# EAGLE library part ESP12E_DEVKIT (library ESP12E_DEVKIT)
ESP12E DEVKIT BOARD
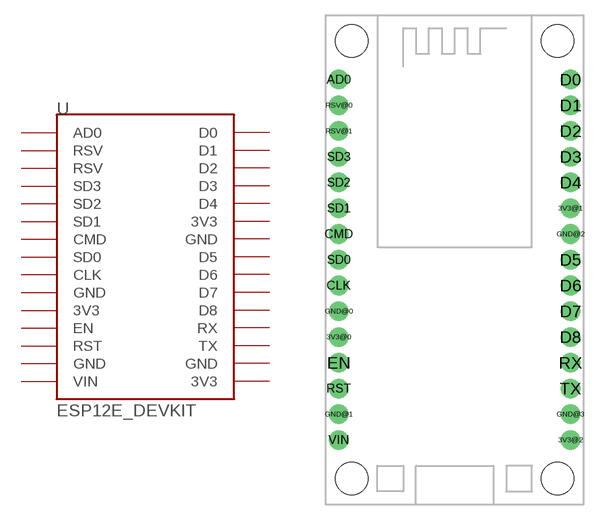
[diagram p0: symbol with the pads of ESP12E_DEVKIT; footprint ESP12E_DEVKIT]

Designator prefix -

## ESP12E_DEVKIT  [ESP12E_DEVKIT]
3V3@0  3V3
3V3@1  3V3
3V3@2  3V3
AD0  AD0
CLK  CLK
CMD  CMD
D0  D0
D1  D1
D2  D2
D3  D3
D4  D4
D5  D5
D6  D6
D7  D7
D8  D8
EN  EN
GND@0  GND
GND@1  GND
GND@2  GND
GND@3  GND
RST  RST
RSV@0  RSV
RSV@1  RSV
RX  RX
SD0  SD0
SD1  SD1
SD2  SD2
SD3  SD3
TX  TX
VIN  VIN

## Footprint ESP12E_DEVKIT (pad centres in mm)
ESP12E_DEVKIT
drill 0.8 pad 1.93: 3V3@0 -11.43,-7.62; 3V3@1 11.43,5.08; 3V3@2 11.43,-17.78; AD0 -11.43,17.78; CLK -11.43,-2.54; CMD -11.43,2.54; D0 11.43,17.78; D1 11.43,15.24; D2 11.43,12.7; D3 11.43,10.16; D4 11.43,7.62; D5 11.43,0; D6 11.43,-2.54; D7 11.43,-5.08; D8 11.43,-7.62; EN -11.43,-10.16; GND@0 -11.43,-5.08; GND@1 -11.43,-15.24; GND@2 11.43,2.54; GND@3 11.43,-15.24; RST -11.43,-12.7; RSV@0 -11.43,15.24; RSV@1 -11.43,12.7; RX 11.43,-10.16; SD0 -11.43,0; SD1 -11.43,5.08; SD2 -11.43,7.62; SD3 -11.43,10.16; TX 11.43,-12.7; VIN -11.43,-17.78
hole 3.2 at -10.16,21.59
hole 3.2 at 10.16,21.59
hole 3.2 at 10.16,-21.59
hole 3.2 at -10.16,-21.59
